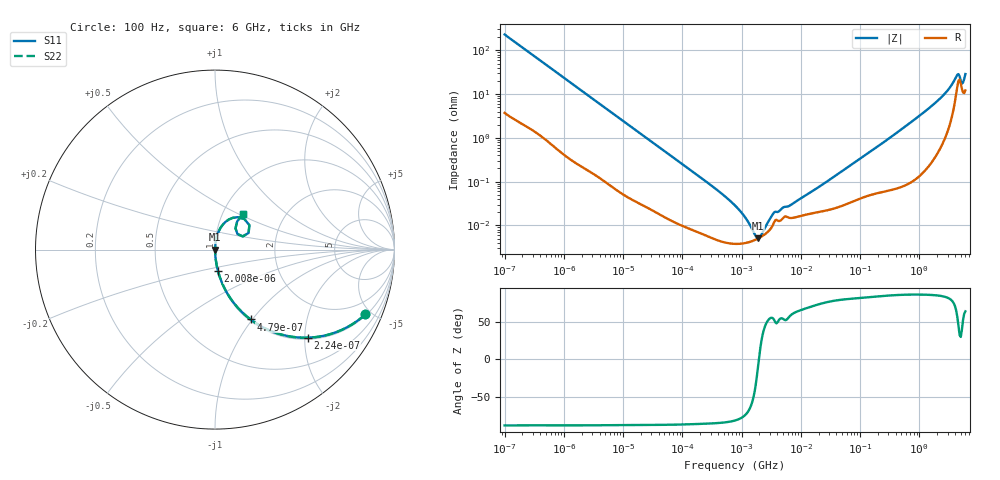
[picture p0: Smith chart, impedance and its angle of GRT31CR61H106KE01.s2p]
!Murata Part Number: GRT31CR61H106KE01
!These Parameters are Measured in Series Mode Connection
!Data Generated on Jun 19, 2026
!  o--ll--o
!Port1  Port2
!  o------o
!Operation Temp=25[degC], DC Bias Voltage=0[V]
!Freq. Start=100[Hz] Stop=6[GHz] 401[Steps]
# Hz S RI R 50
!Freq.(Hz) S11(Real) S11(Imag) S21(Real) S21(Imag) S12(Real) S12(Imag) S22(Real) S22(Imag)
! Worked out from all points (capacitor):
!   401 points, 100 Hz to 6 GHz, reference 50 ohm
!   read as one part in series: C = 6.88 uF near 109 Hz
!   lowest |Z| = 5.09 mohm at 1.897 MHz (marker M1)
!   series resonance near 1.959 MHz, so ESL is about 960 pH
!   S11 on the Smith chart (normalised r, x): 100 Hz: 1.07, -4.61; 224 Hz: 1.04, -2.07; 479 Hz: 1.02, -0.98; 2.008 kHz: 1.00, -0.24; 6 GHz: 1.24, +0.52
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100  0.8376 -0.3608  0.1624 0.3608  0.1624 0.3608  0.8376 -0.3608
224  0.5181 -0.4907  0.4819 0.4907  0.4819 0.4907  0.5181 -0.4907
479  0.1981 -0.3892  0.8019 0.3892  0.8019 0.3892  0.1981 -0.3892
897  0.0688 -0.2444  0.9312 0.2444  0.9312 0.2444  0.0688 -0.2444
2008  0.016 -0.1165  0.984 0.1165  0.984 0.1165  0.016 -0.1165
6433  0.00217 -0.0375  0.9978 0.0375  0.9978 0.0375  0.00217 -0.0375
40335  0.000219 -0.00614  0.9998 0.00614  0.9998 0.00614  0.000219 -0.00614
330837  5.04e-05 -0.000758  0.9999 0.000758  0.9999 0.000758  5.04e-05 -0.000758
774597  3.79e-05 -0.000283  1 0.000283  1 0.000283  3.79e-05 -0.000283
1386327  4.21e-05 -9.29e-05  1 9.29e-05  1 9.29e-05  4.21e-05 -9.29e-05
1896632  5.02e-05 -8.4e-06  0.9999 8.4e-06  0.9999 8.4e-06  5.02e-05 -8.4e-06
2481164  6.29e-05 6.21e-05  0.9999 -6.21e-05  0.9999 -6.21e-05  6.29e-05 6.21e-05
3549919  0.000118 0.000159  0.9999 -0.000159  0.9999 -0.000159  0.000118 0.000159
6644369  0.000148 0.000247  0.9999 -0.000247  0.9999 -0.000247  0.000148 0.000247
1.555665e7  0.000189 0.000573  0.9998 -0.000573  0.9998 -0.000573  0.000189 0.000573
3.124326e8  0.000725 0.00982  0.9993 -0.00982  0.9993 -0.00982  0.000725 0.00982
1.873145e9  0.00766 0.0628  0.9923 -0.0628  0.9923 -0.0628  0.00766 0.0628
3.205649e9  0.0348 0.1272  0.9652 -0.1272  0.9652 -0.1272  0.0348 0.1272
4.193612e9  0.1288 0.1806  0.8712 -0.1806  0.8712 -0.1806  0.1288 0.1806
4.586474e9  0.1916 0.1363  0.8084 -0.1363  0.8084 -0.1363  0.1916 0.1363
5.245841e9  0.125 0.0872  0.875 -0.0872  0.875 -0.0872  0.125 0.0872
6e9  0.1539 0.1963  0.8461 -0.1963  0.8461 -0.1963  0.1539 0.1963
